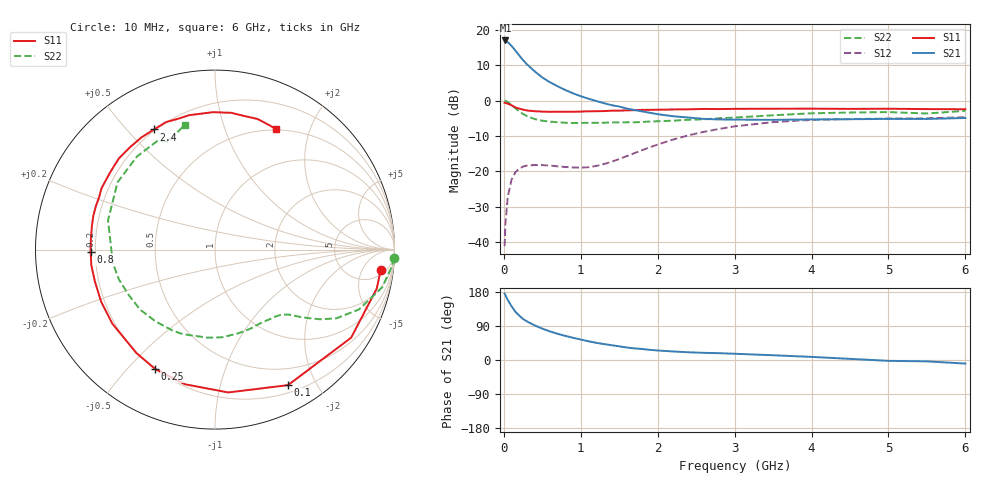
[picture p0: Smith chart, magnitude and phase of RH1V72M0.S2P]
! SIEMENS Small Signal Semiconductors
! BFR106
! Si NPN RF Bipolar Junction Transistor in SOT23
! VCE = 1.75 V  IC = 2 mA
! Common Emitter S-Parameters:  August  1996
# GHz  S  MA  R  50
!  f  S11  S21  S12  S22
! GHz  MAG  ANG  MAG  ANG  MAG  ANG  MAG  ANG
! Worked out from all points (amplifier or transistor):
!   36 points, 10 MHz to 6 GHz, reference 50 ohm
!   highest |S21| = 17.0 dB at 20 MHz (marker M1)
!   |S21| within 3 dB of that: start of sweep to 154.4 MHz
!   unconditionally stable (mu >= 1): 772.3 MHz to 2.454 GHz; 2.657 GHz to end of sweep
!   at 250 MHz: K = 0.33, MSG = 15.1 dB, |S12| = -18.7 dB
!   at 1.4 GHz: K = 1.31, MAG = 4.7 dB, |S12| = -17.3 dB
!   at 6 GHz: K = 1.02, MAG = -1.1 dB, |S12| = -4.7 dB
!   S11 on the Smith chart (normalised r, x): 10 MHz: 7, -12; 100 MHz: 0.29, -1.64; 250 MHz: 0.20, -0.60; 800 MHz: 0.18, -0.01; 2.4 GHz: 0.19, +0.60; 6 GHz: 0.49, +1.51
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0.01  0.9303 -6.9  7.062 175.1  0.0087 88.9  0.9977 -2.6
0.02  0.927 -13.5  7.078 171.5  0.0177 82.8  0.991 -5.3
0.05  0.9035 -32.9  6.704 158.8  0.0427 71.3  0.9544 -12.8
0.1  0.8577 -61.7  5.933 141.9  0.0757 57.6  0.8683 -22.6
0.15  0.7993 -84.7  5.08 127.2  0.0968 45.6  0.7761 -29.6
0.2  0.7687 -102.6  4.352 117.1  0.1087 38.4  0.7032 -33.5
0.25  0.7439 -116.6  3.732 108.2  0.1164 32.4  0.643 -36.4
0.3  0.7238 -127.2  3.261 101.9  0.1201 29.0  0.603 -38.4
0.4  0.7054 -144.2  2.591 91.4  0.1224 24.1  0.5469 -41.4
0.5  0.6976 -155.5  2.119 82.8  0.122 21.7  0.5181 -44.4
0.6  0.6923 -165.2  1.813 75.4  0.1203 21.0  0.5028 -47.9
0.8  0.6932 -179.0  1.407 63.6  0.1147 24.6  0.485 -55.9
1.1  0.7034 164.8  1.062 49.4  0.1138 37.3  0.4829 -69.8
1.6  0.7252 143.8  0.768 32.9  0.1639 57.9  0.4924 -95.7
2.2  0.7475 123.2  0.6 22.5  0.2804 58.2  0.5189 -129.2
2.4  0.751 116.9  0.574 20.4  0.3218 55.0  0.5344 -141.1
3  0.7626 100.9  0.537 16.5  0.431 42.0  0.5742 -172.6
3.5  0.7658 90.9  0.533 12.5  0.4952 30.7  0.6181 164.6
4.5  0.7619 77.0  0.544 3.0  0.5472 11.1  0.6768 130.0
5  0.7654 71.9  0.55 -2.2  0.5551 3.9  0.6862 117.6
5.5  0.7566 66.7  0.549 -3.6  0.5609 0.5  0.6554 113.5
6  0.7532 63.3  0.566 -9.4  0.5822 -6.9  0.7149 103.7
